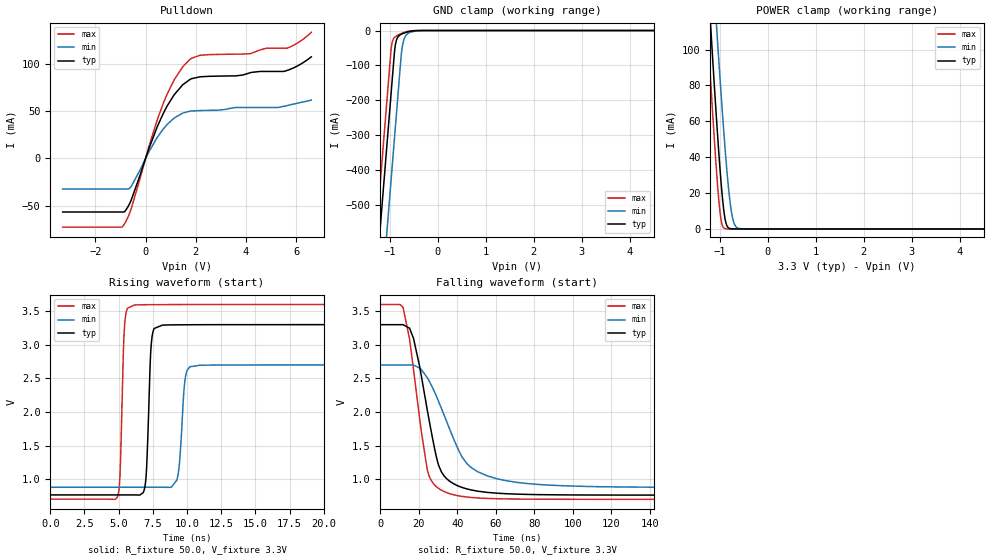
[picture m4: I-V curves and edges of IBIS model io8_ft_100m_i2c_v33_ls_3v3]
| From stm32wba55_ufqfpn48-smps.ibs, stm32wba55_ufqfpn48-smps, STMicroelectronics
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[Model]   io8_ft_100m_i2c_v33_ls_3v3
Model_type I/O_open_drain
Polarity   Non-Inverting
Enable   Active-Low
| CAP_THRESHOLD on pad IOFT is "UDTCAPC" :
| Rising=30.0% of vddiom   Falling=70.0% of vddiom
| C_comp min and max val. don't necessarily correlate with the min and max pvt
| but are the smallest and greatest pad capacitance found.
| var   typ   min   max
C_comp   2.70467pF  2.60096pF  2.73929pF
|C_comp_pulldown   2.70467pF  2.60096pF  2.73929pF
Vinl = 1.35V
Vinh = 1.8V
Vmeas = 1.65V   | Reference voltage for timing measurements
Cref  = 50.0pF   | Timing specification test load capacitance value
Rref  = 1.0MOhm   | Timing specification test load resistance value
Vref  = 1.815V   | Timing specification test load voltage
[Model Spec]
| TIME_THRESHOLD on pin ZII2CV11 is "CMOS" :
| Rising=50.0% of vdd   Falling=50.0% of vdd
Vinl 1.28450V 1.07650V 1.38450V
Vinh 1.79550V 1.49050V 1.94250V
| variable   typ   min   max
[Temperature Range] 25.0 140.0 -40.0
| variable   typ   min   max
[Voltage Range] 3.3V 2.7V 3.6V
| variable   typ   min   max
[POWER Clamp Reference] 3.3V 2.7V 3.6V
| variable   typ   min   max
[GND Clamp Reference] 0V 0V 0V
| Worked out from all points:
|   slope of the pulldown table from 0 to 0.495 V, typ, clamps not added: 14 ohm
|   GND clamp passes 1 mA (typ) near -0.51 V on its own axis
|   POWER clamp passes 1 mA (typ) near -0.83 V on its own axis
|   rising waveform, R_fixture 50.0, V_fixture 3.3V: 20-80 % time 255ps typ, 332ps min, 231ps max; typ from 0.764 V to 3.3 V
|   falling waveform, R_fixture 50.0, V_fixture 3.3V: 20-80 % time 10.1ns typ, 17.2ns min, 8.14ns max; typ from 3.3 V to 0.764 V
[POWER Clamp]
-3.3V     1.123A     1.139A     1.091A
-1.36V    189.2mA    238.8mA    158.1mA
-1.25V    139mA      190.3mA    108.1mA
-1.18V    107.9mA    159.9mA    77.22mA
-1.06V    57.23mA    109.3mA    28.68mA
-980mV    27.6mA     77.28mA    5.935mA
-900mV    6.895mA    47.74mA    242.8uA
-820mV    594.6uA    22.85mA    5.912uA
-760mV    69.41uA    9.714mA    358.6nA
-700mV    7.83uA     2.919mA    21.86nA
-630mV    611.5nA    529.9uA    954.5pA
6.6V      0A         0A         0A
[GND Clamp]
-3.3V     -4.134A    -4.382A    -4.006A
-1.59V    -1.227A    -1.475A    -1.099A
-1.25V    -648.9mA   -896.7mA   -520.9mA
-980mV    -189.9mA   -437.7mA   -61.92mA
-970mV    -172.9mA   -420.7mA   -48.45mA
-910mV    -70.86mA   -318.7mA   -21.03mA
-880mV    -37.23mA   -267.7mA   -17.31mA
-750mV    -9.908mA   -55.25mA   -7.768mA
-710mV    -7.626mA   -27.41mA   -5.608mA
-650mV    -4.885mA   -11.6mA    -3.058mA
-360mV    -31.22uA   -443.6uA   -1.188uA
6.6V      2.31nA     2.655uA    974.6pA
| variable   typ   min   max
[Pullup Reference] 3.3V 2.7V 3.6V
| variable   typ   min   max
[Pulldown Reference] 0V 0V 0V
[Pulldown]
-3.3V     -56.7mA    -32.4mA    -72.73mA
-890mV    -56.7mA    -32.4mA    -71.32mA
-570mV    -43.94mA   -29.54mA   -52.99mA
120mV     9.474mA    6.407mA    11.48mA
700mV     47.33mA    30.97mA    57.88mA
1.14V     67.41mA    42.74mA    83.2mA
1.78V     83.75mA    50.04mA    105.1mA
2.17V     86.37mA    50.65mA    109.1mA
4.16V     90.61mA    53.89mA    110.8mA
4.82V     92.03mA    53.89mA    116.6mA
5.63V     93.04mA    55.89mA    116.6mA
6.6V      107.5mA    61.71mA    133.4mA
[Ramp]
dV/dt_r 1.52155V/251.23804ps 1.09308V/330.45414ps 1.73921V/226.7151ps
dV/dt_f 1.52157V/9.99291ns 1.09311V/17.14718ns 1.73923V/7.98689ns
R_load = 50.0
| Removed startup time: 0s 0s 0s  .
| Removed end time: 33.35ns.
[Rising Waveform]
R_fixture   = 50.0
V_fixture   = 3.3V
V_fixture_min = 2.7V
V_fixture_max = 3.6V
0s        764mV      878.1mV    701.3mV
4.9ns     764mV      878.1mV    727.3mV
5.1ns     764mV      878.1mV    1.058V
5.45ns    764mV      878.1mV    3.329V
6.15ns    764mV      878.1mV    3.592V
6.95ns    923.1mV    878.1mV    3.597V
7.6ns     3.243V     878.1mV    3.598V
9.25ns    3.297V     982.8mV    3.599V
10.2ns    3.298V     2.672V     3.599V
33.35ns   3.3V       2.7V       3.6V
| Removed startup time: 0s 0s 0s  .
| Removed end time: 248.4ns.
[Falling Waveform]
R_fixture   = 50.0
V_fixture   = 3.3V
V_fixture_min = 2.7V
V_fixture_max = 3.6V
0s        3.3V       2.7V       3.6V
11.8ns    3.3V       2.7V       3.56V
15.2ns    3.248V     2.7V       3.09V
20.3ns    2.697V     2.656V     1.932V
24.4ns    2.032V     2.512V     1.143V
29.8ns    1.255V     2.191V     874.8mV
34.55ns   1.006V     1.853V     800.5mV
45.65ns   851.8mV    1.215V     733.6mV
65.9ns    784.1mV    975.4mV    707.3mV
248.4ns   764mV      878.1mV    701.3mV
